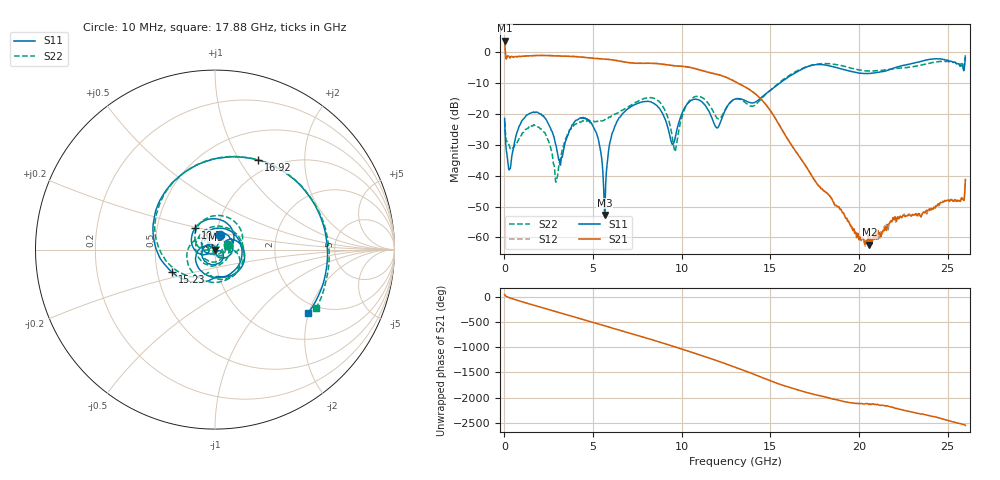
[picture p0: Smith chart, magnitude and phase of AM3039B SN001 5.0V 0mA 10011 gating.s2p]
!Agilent Technologies,E8364B,MY43040894,A.07.50.67
!Agilent E8364B: A.07.50.67
!Date: Tuesday, June 28, 2016 08:08:07
!Correction: S11(Full 2 Port(1,2))
!S21(Full 2 Port(1,2))
!S12(Full 2 Port(1,2))
!S22(Full 2 Port(1,2))
!S2P File: Measurements: S11, S21, S12, S22:
# Hz S  dB  R 50
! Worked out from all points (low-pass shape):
!   1601 points, 10 MHz to 26 GHz, reference 50 ohm
!   highest |S21| = 3.72 dB at 10 MHz (marker M1); lowest = -62.3 dB at 20.59 GHz (marker M2)
!   |S21| within 3 dB of the highest: start of sweep to 44.04 MHz
!   lowest |S11| = -52.7 dB at 5.663 GHz (marker M3), VSWR 1.00, Z = 50.2 - j0.038 ohm
!   |S11| at or under -10 dB: start of sweep to 15.53 GHz
!   |S22| runs from -42.1 to -1.0 dB; largest |S21 - S12| = 0.025
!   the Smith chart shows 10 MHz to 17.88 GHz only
!   S11 on the Smith chart (normalised r, x): 10 MHz: 1.05, +0.17; 10.5 GHz: 0.78, +0.19; 15.23 GHz: 0.60, -0.16; 16.92 GHz: 0.84, +1.21; 17.88 GHz: 1.71, -1.99
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1e7  -21.42 70.0  3.72 40.9  3.79 41.7  -22.40 20.2
7.24725e8  -25.82 137.9  -1.55 -73.6  -1.50 -73.4  -29.16 -173.6
1.683106e9  -19.51 41.1  -1.13 -172.8  -1.09 -172.6  -23.62 38.1
2.73895e9  -26.55 -65.0  -1.16 80.2  -1.10 80.4  -35.22 -122.2
3.534894e9  -27.49 -22.6  -1.34 -0.3  -1.27 -0.1  -26.97 -11.1
4.347081e9  -21.33 -108.9  -1.61 -83.5  -1.58 -83.4  -22.46 -134.7
5.662825e9  -52.70 -9.4  -2.25 141.2  -2.21 141.4  -21.87 -25.0
7.011056e9  -18.21 75.7  -3.40 1.7  -3.35 1.8  -17.58 83.3
8.684162e9  -17.83 -144.3  -3.75 -173.5  -3.69 -173.3  -15.80 -164.9
9.610056e9  -28.30 -156.6  -4.44 85.7  -4.38 85.8  -32.23 145.9
1.050346e10  -15.74 132.7  -4.98 -16.0  -4.93 -16.0  -15.32 117.0
1.181921e10  -23.04 14.3  -6.99 -169.0  -6.93 -169.1  -19.72 -10.7
1.3005e10  -15.19 -20.3  -9.56 42.8  -9.51 42.7  -15.21 -49.0
1.523039e10  -11.36 -152.4  -20.99 101.6  -20.89 101.5  -11.18 -165.1
1.691974e10  -5.12 64.2  -36.22 -85.8  -36.14 -85.9  -4.94 57.9
1.734208e10  -4.27 21.4  -40.07 -127.1  -40.04 -127.2  -4.19 19.4
1.787812e10  -4.03 -34.1  -44.20 -168.2  -44.17 -169.5  -3.73 -29.9
2.059083e10  -6.91 98.2  -62.34 26.8  -60.52 39.6  -6.10 109.3
2.167916e10  -5.71 23.6  -55.71 -13.6  -56.32 -12.7  -5.62 31.2
2.320608e10  -3.36 -91.7  -52.31 -145.3  -53.05 -144.6  -4.53 -80.2
2.432689e10  -2.14 177.5  -49.86 135.5  -50.20 135.3  -3.17 -165.6
2.6e10  -1.85 -13.4  -41.27 -31.7  -41.30 -32.5  -0.99 19.8
